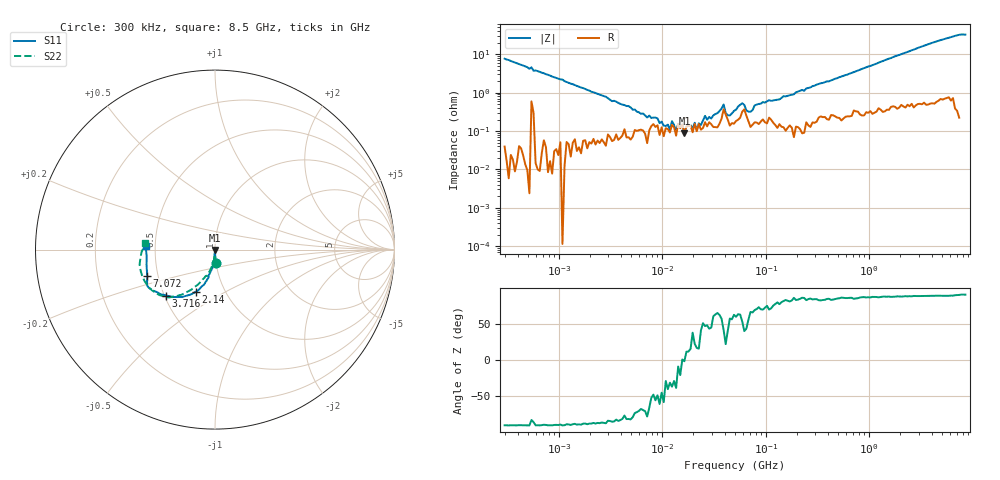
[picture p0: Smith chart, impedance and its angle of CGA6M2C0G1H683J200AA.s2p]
! S-parameter Generated by TDK Corporation
! Copyright(C) 2015 TDK Corporation.
! All Rights Reserved.
! TDK P/N: CGA6M2C0G1H683J200AA (Multilayer Ceramic Chip Capacitors)
! Property: C=68nF
! Size(LxWxT): 3.2x2.5x2mm, 0.126x0.098x0.079inches
! Model Type: s2p (Touchstone File Format Version 1.0)
! Frequency: DC=Yes Start=0.3MHz Stop=8500MHz 225points Log-sweep
! Note:
! Model Generated on Jun. 23, 2015
! Hash(MD5):
! Port Assignments:
!  1 ---| |--- 2
! Applicable Conditions:
!  Temperature = 25 degC
!  DC Bias Voltage = 0 V
!  Small Signal Operation
! Terms and conditions regarding TDK Simulation Models
! (1)This simulation model is being provided solely for informational purposes. Please refer to the specifications of the products in terms of detailed characteristics of such products.
! (2)In no event shall TDK Corporation of any of its subsidiaries be liable for any loss or damage arising, directly or indirectly,
!  From any information contained in this simulation model, including, but not limited to loss or damages arising from any inaccuracies, omissions or errors in connection with such information.
! (3)Any and all copyrights on this simulation model are owned by TDK Corporation.
!  Duplication or redistribution of this simulation model without prior written permission from TDK Corporation is prohibited.
! (4)This simulation model is subject to any modification or change without any prior notice.
! (5)Neither TDK Corporation nor any of its subsidiaries shall make any warranty, express or implied,
!  Including but not limited to the correctness, implied warranties of merchantability and fitness for a particular purpose with respect to this simulation models.
! (6)The use of this simulation model shall be deemed to have consented to the terms and conditions hereof.
# MHz S MA R 50
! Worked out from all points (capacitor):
!   224 points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, 300 kHz to 8.5 GHz, reference 50 ohm
!   read as one part in series: C = 69 nF near 314.1 kHz
!   lowest |Z| = 86.9 mohm at 16.37 MHz (marker M1)
!   series resonance near 15.61 MHz, so ESL is about 1.5 nH
!   S11 on the Smith chart (normalised r, x): 300 kHz: 1.00, -0.15; 2.14 GHz: 0.73, -0.37; 3.716 GHz: 0.51, -0.30; 7.072 GHz: 0.44, -0.15; 8.5 GHz: 0.44, +0.02
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0.3  0.07598 -86.0  0.9968 4.3  0.9965 4.5  0.07666 -84.9
1.72111  0.01287 -87.7  0.9994 0.7  0.9989 0.8  0.01304 -87.8
4.954665  0.004589 -83.1  0.9996 0.1  0.9992 0.3  0.00464 -82.0
9.430415  0.002925 -76.2  0.9995 -0.0  0.9988 0.0  0.003172 -76.0
16.37255  0.0026 -74.7  0.9992 -0.2  0.999 -0.1  0.003189 -72.0
29.76236  0.003024 -73.5  0.9983 -0.4  0.9979 -0.3  0.004406 -72.5
37.45369  0.002819 -58.4  0.9978 -0.6  0.9974 -0.5  0.004826 -64.1
39.21571  0.004519 -49.3  0.9961 -0.7  0.9957 -0.6  0.006314 -56.1
41.06062  0.005587 -68.3  0.9971 -0.5  0.9968 -0.4  0.007607 -70.1
45.01492  0.004951 -84.1  0.9984 -0.6  0.998 -0.5  0.007207 -79.1
51.67171  0.004997 -86.9  0.9972 -0.7  0.997 -0.7  0.007296 -81.1
56.64789  0.005038 -79.0  0.9968 -0.9  0.9971 -0.8  0.007395 -76.6
65.02496  0.008347 -81.2  0.9973 -0.8  0.9961 -0.8  0.01095 -79.4
81.82903  0.008956 -91.3  0.9976 -1.2  0.9963 -1.1  0.0116 -87.5
283.1228  0.03701 -95.2  0.9938 -3.8  0.9958 -3.7  0.03487 -96.1
469.456  0.06335 -95.6  0.9934 -6.5  0.993 -6.2  0.06562 -96.7
1551.304  0.1962 -106.9  0.9732 -20.5  0.972 -20.2  0.1934 -114.0
2140.204  0.258 -114.7  0.955 -28.0  0.9546 -27.5  0.2615 -120.8
3715.7  0.3751 -137.0  0.9124 -46.3  0.9098 -46.0  0.377 -135.2
5367.404  0.4268 -150.5  0.8847 -63.2  0.8846 -62.6  0.4262 -152.5
7072.242  0.4051 -158.9  0.8842 -79.3  0.8799 -78.9  0.4099 -178.0
8500  0.3866 177.4  0.888 -95.8  0.8907 -95.1  0.3901 174.7
